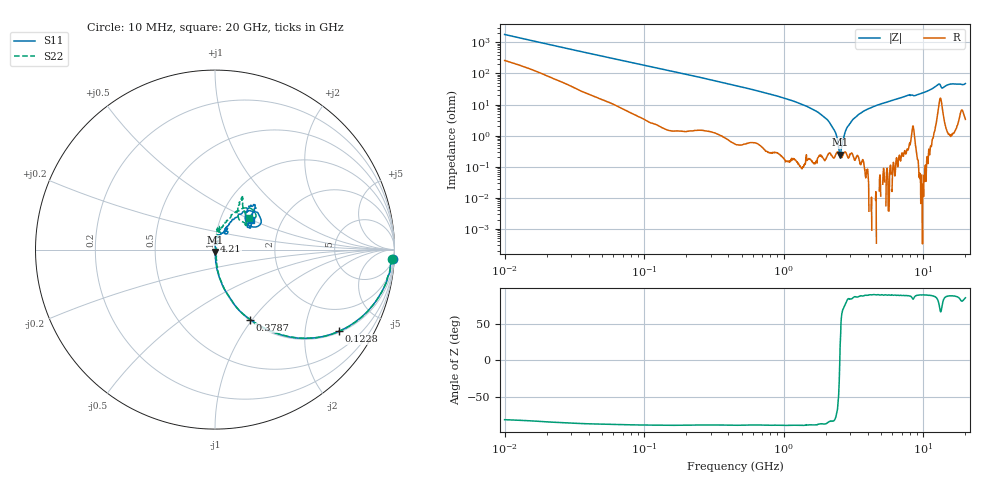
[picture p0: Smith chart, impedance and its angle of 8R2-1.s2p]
!Keysight Technologies,P5008B,MY61100088,A.16.20.02
!Date: Monday, May 27, 2024 16:46:58
!Correction: S11(C* 2-Port  )
!S21(C* 2-Port  )
!S12(C* 2-Port  )
!S22(C* 2-Port  )
!S2P File: Measurements: S11, S21, S12, S22:Log Frequency Sweep
# Hz S  dB  R 50
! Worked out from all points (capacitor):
!   1601 points, 10 MHz to 20 GHz, reference 50 ohm
!   read as one part in series: C = 8.99 pF near 10.39 MHz
!   lowest |Z| = 243 mohm at 2.521 GHz (marker M1)
!   series resonance near 2.52 GHz, so ESL is about 440 pH
!   S11 on the Smith chart (normalised r, x): 10 MHz: 5, -36; 122.8 MHz: 1.05, -3.02; 378.7 MHz: 1.01, -0.98; 4.21 GHz: 0.99, +0.09; 20 GHz: 1.40, +0.49
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1e7  -0.07 -3.1  -25.16 78.5  -25.17 78.5  -0.09 -3.1
3.555162e7  -0.25 -11.1  -14.27 75.8  -14.28 75.9  -0.26 -11.1
1.2284e8  -1.64 -33.2  -5.24 55.9  -5.25 55.9  -1.63 -33.3
1.263918e8  -1.71 -34.0  -5.07 55.2  -5.09 55.2  -1.70 -34.0
3.787084e8  -7.21 -63.3  -0.99 25.7  -1.00 25.7  -7.20 -63.4
4.472136e8  -8.39 -67.2  -0.73 22.1  -0.74 22.1  -8.38 -67.2
9.076605e8  -14.57 -79.1  -0.17 10.2  -0.18 10.2  -14.59 -78.8
1.589917e9  -22.06 -85.9  -0.03 3.7  -0.04 3.7  -21.91 -83.3
2.054869e9  -27.35 -86.4  -0.01 1.2  -0.02 1.2  -26.97 -80.3
2.347211e9  -31.82 -85.2  0.00 -0.1  -0.01 -0.1  -31.23 -75.3
2.520573e9  -37.51 -79.8  0.00 -0.8  -0.01 -0.8  -35.88 -65.8
2.865525e9  -51.99 46.3  0.00 -2.1  -0.01 -2.1  -43.13 19.5
3.211587e9  -36.48 87.7  0.01 -3.3  -0.01 -3.3  -34.04 65.7
3.633803e9  -30.37 89.9  0.01 -4.6  -0.01 -4.6  -28.60 71.0
4.210356e9  -26.43 95.1  0.01 -6.2  -0.01 -6.2  -25.44 71.2
5.652411e9  -22.02 78.2  -0.01 -9.9  -0.02 -9.9  -22.08 80.4
7.697294e9  -17.78 61.3  -0.06 -15.2  -0.06 -15.3  -18.02 81.1
9.264046e9  -18.91 62.4  -0.03 -18.3  -0.04 -18.3  -18.83 77.2
1.273595e10  -10.40 44.7  -0.84 -30.2  -0.84 -30.2  -10.54 51.7
1.380717e10  -12.43 45.1  -0.62 -24.9  -0.64 -24.9  -12.82 56.0
1.592205e10  -9.58 48.2  -0.51 -32.5  -0.52 -32.5  -9.71 61.3
2e10  -11.81 39.4  -0.52 -40.2  -0.53 -40.2  -11.77 43.4
